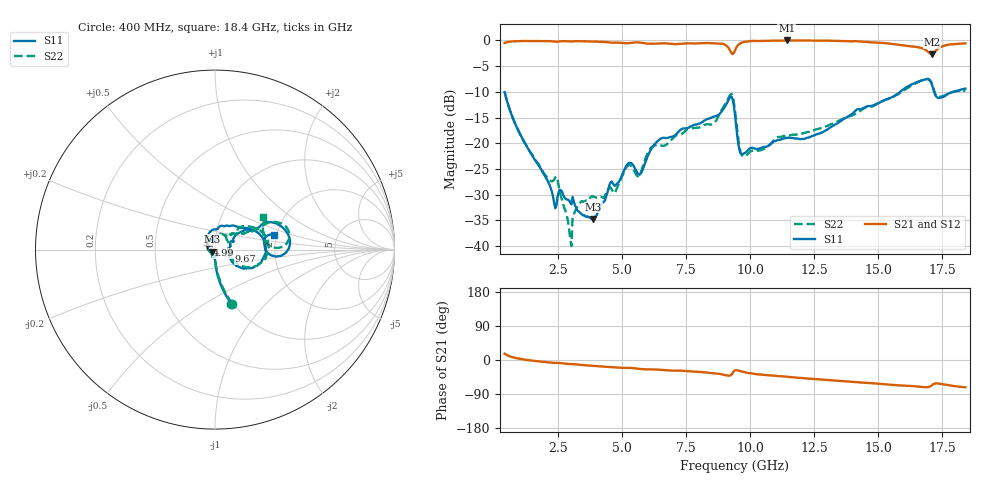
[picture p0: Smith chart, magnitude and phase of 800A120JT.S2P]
!  American Technical Ceramics  Date:  12/17/08
!  One Norden Lane
!  Huntington Station,  NY.  11746-2102
!  Tel:  (631) 622-4700  Fax:  (631) 622-4748
!  Part Number  800A120JT
!  Description: Broardband capacitor  Mounting Orientation: Vertical
!  Application:
# GHZ S DB R 50
! Freq  |S11|  S11 Ph  |S21|  S21 Ph  |S12|  S12 Ph  |S22|  S22 Ph
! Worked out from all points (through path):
!   401 points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, 400 MHz to 18.4 GHz, reference 50 ohm
!   highest |S21| = 0.00 dB at 11.43 GHz (marker M1); lowest = -2.7 dB at 17.09 GHz (marker M2)
!   group delay of S21, straight-line fit = 11.8 ps
!   lowest |S11| = -34.7 dB at 3.865 GHz (marker M3), VSWR 1.04, Z = 48.5 - j1.05 ohm
!   |S11| at or under -10 dB: start of sweep to 15.85 GHz; 17.18 GHz to 17.93 GHz (749.9 MHz wide, 4.27 % of centre)
!   |S22| runs from -40.0 to -7.5 dB; largest |S21 - S12| = 0.0038
!   S11 on the Smith chart (normalised r, x): 400 MHz: 0.98, -0.66; 4.99 GHz: 0.92, +0.05; 9.67 GHz: 1.17, -0.02; 18.4 GHz: 1.94, +0.36
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0.4  -10.04 -73.2  -0.49 16.7  -0.47 16.7  -10.02 -72.3
1.255  -20.52 -87.4  -0.10 0.3  -0.09 0.2  -20.52 -86.4
2.335  -31.55 -87.5  -0.21 -7.7  -0.19 -7.7  -27.06 -89.4
2.92  -31.17 -91.3  -0.19 -10.5  -0.17 -10.6  -36.78 -125.3
3.415  -33.80 -118.4  -0.15 -13.2  -0.14 -13.2  -31.21 -111.3
3.865  -34.74 -143.7  -0.21 -15.6  -0.20 -15.7  -30.38 -139.3
4.72  -28.28 154.2  -0.40 -19.5  -0.39 -19.6  -29.51 165.0
4.99  -26.13 147.9  -0.50 -20.7  -0.49 -20.8  -26.39 146.6
5.305  -23.77 121.5  -0.49 -20.8  -0.49 -20.9  -24.25 104.7
5.71  -25.94 117.4  -0.43 -23.8  -0.42 -23.9  -25.80 93.4
6.43  -19.35 100.4  -0.57 -25.5  -0.57 -25.6  -20.38 55.8
8.545  -14.86 44.0  -0.55 -34.7  -0.56 -34.9  -16.21 38.2
9.22  -10.96 6.3  -2.06 -40.7  -2.08 -40.9  -10.51 10.6
9.4  -14.48 -34.2  -1.92 -27.4  -1.94 -27.5  -13.62 -28.6
9.67  -22.14 -6.2  -0.42 -30.7  -0.43 -30.9  -22.37 -4.9
11.425  -18.96 24.5  0.00 -44.1  -0.01 -44.2  -18.53 46.5
12.415  -18.58 30.1  -0.01 -49.7  -0.02 -49.8  -17.54 41.2
15.43  -11.25 26.9  -0.61 -65.1  -0.62 -65.1  -11.26 25.5
16.465  -8.20 19.8  -1.24 -69.5  -1.25 -69.5  -8.32 23.1
17.095  -8.60 -5.3  -2.70 -66.5  -2.72 -66.5  -8.48 2.2
17.365  -11.16 5.8  -1.46 -62.3  -1.47 -62.2  -11.04 15.2
18.4  -9.36 14.1  -0.57 -72.1  -0.58 -72.0  -9.82 34.5
